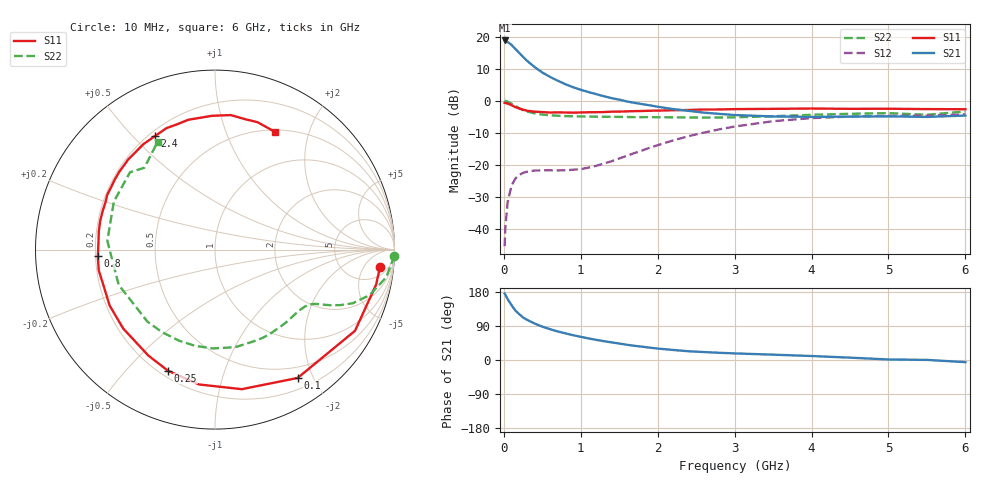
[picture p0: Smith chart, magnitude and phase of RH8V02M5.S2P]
! SIEMENS Small Signal Semiconductors
! BFR106
! Si NPN RF Bipolar Junction Transistor in SOT23
! VCE = 8 V  IC = 2.5 mA
! Common Emitter S-Parameters:  August  1996
# GHz  S  MA  R  50
!  f  S11  S21  S12  S22
! GHz  MAG  ANG  MAG  ANG  MAG  ANG  MAG  ANG
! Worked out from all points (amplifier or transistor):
!   36 points, 10 MHz to 6 GHz, reference 50 ohm
!   highest |S21| = 18.8 dB at 10 MHz (marker M1)
!   |S21| within 3 dB of that: start of sweep to 163.7 MHz
!   unconditionally stable (mu >= 1): 752.4 MHz to 1.829 GHz; 4.335 GHz to end of sweep
!   at 250 MHz: K = 0.35, MSG = 18.1 dB, |S12| = -22.5 dB
!   at 1.4 GHz: K = 1.20, MAG = 7.1 dB, |S12| = -18.9 dB
!   at 6 GHz: K = 1.02, MAG = -1.0 dB, |S12| = -4.2 dB
!   S11 on the Smith chart (normalised r, x): 10 MHz: 9, -12; 100 MHz: 0.34, -1.78; 250 MHz: 0.23, -0.66; 800 MHz: 0.21, -0.03; 2.4 GHz: 0.22, +0.58; 6 GHz: 0.52, +1.50
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0.01  0.9243 -6.1  8.678 175.3  0.0054 88.9  0.9978 -1.9
0.02  0.9186 -12.3  8.597 172.3  0.0106 84.6  0.9897 -3.9
0.05  0.9018 -30.1  8.192 160.4  0.0265 74.0  0.9661 -9.2
0.1  0.8505 -57.2  7.415 144.7  0.0475 61.0  0.8981 -16.4
0.15  0.792 -79.1  6.383 130.6  0.0611 50.1  0.8231 -21.3
0.2  0.7566 -96.8  5.553 120.9  0.0697 44.1  0.7635 -23.9
0.25  0.7237 -111.3  4.816 112.2  0.075 38.2  0.7121 -25.8
0.3  0.6974 -122.2  4.197 106.2  0.0781 35.6  0.678 -26.9
0.4  0.6745 -139.3  3.342 96.3  0.0814 31.7  0.6331 -28.5
0.5  0.6647 -152.1  2.746 88.0  0.0821 30.7  0.6072 -30.2
0.6  0.6526 -161.8  2.351 81.4  0.0822 31.8  0.5923 -32.5
0.8  0.654 -176.7  1.806 70.4  0.0823 37.5  0.5748 -37.6
1.1  0.6595 165.9  1.363 57.0  0.0905 51.6  0.5656 -46.9
1.6  0.6811 145.0  0.972 40.2  0.1384 69.2  0.5562 -65.2
2.2  0.7099 124.2  0.74 26.5  0.2401 70.0  0.5507 -91.5
2.4  0.7156 117.8  0.694 23.1  0.2794 67.2  0.5474 -101.9
3  0.7386 101.6  0.597 17.4  0.3955 55.4  0.5503 -133.1
3.5  0.7456 91.3  0.568 14.1  0.4788 43.8  0.5715 -159.9
4.5  0.7458 76.9  0.564 6.2  0.5652 21.1  0.6238 154.6
5  0.7482 71.5  0.57 1.4  0.5813 12.2  0.6402 137.7
5.5  0.739 66.3  0.558 0.3  0.5819 7.8  0.6024 130.8
6  0.7357 63.2  0.586 -5.7  0.6131 -0.5  0.6796 118.1
